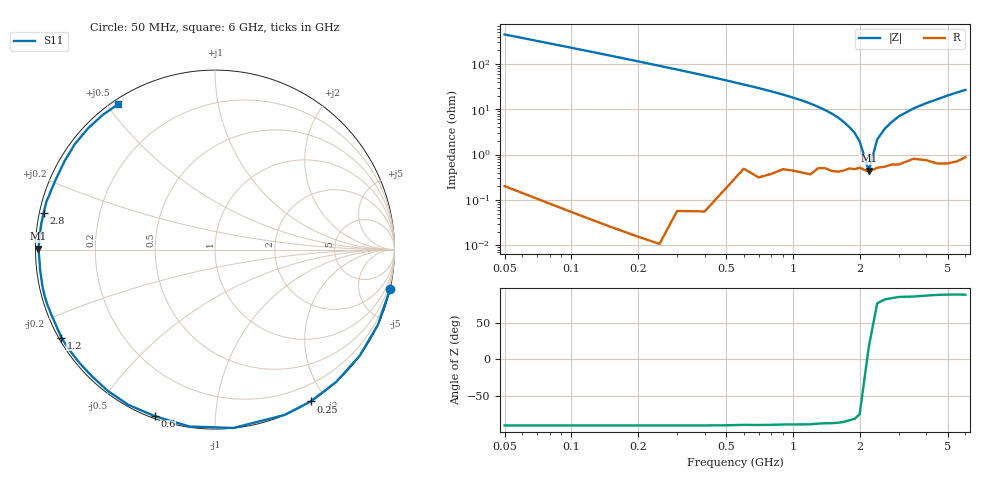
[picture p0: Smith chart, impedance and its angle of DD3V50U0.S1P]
! Infineon Technologies  Discrete & RF Semiconductors
! BBY58-02W
! Si Tuning Diode in SCD-80
! VR = 3.5 V
! S-Parameters:  June  2000
# GHz  S  MA  R  50
!  f  S11
! GHz  MAG  ANG
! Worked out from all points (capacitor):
!   34 points, 50 MHz to 6 GHz, reference 50 ohm
!   read as one part to ground: C = 6.98 pF near 50 MHz
!   lowest |Z| = 438 mohm at 2.2 GHz (marker M1)
!   series resonance near 2.187 GHz, so ESL is about 760 pH
!   S11 on the Smith chart (normalised r, x): 50 MHz: 0.00, -8.92; 250 MHz: 0.00, -1.81; 600 MHz: 0.01, -0.70; 1.2 GHz: 0.01, -0.27; 2.8 GHz: 0.01, +0.11; 6 GHz: 0.02, +0.53
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0.05  0.9999 -12.8
0.1  0.9999 -24.8
0.15  0.9999 -36.4
0.2  0.9999 -47.4
0.25  0.9999 -57.8
0.3  0.9993 -67.3
0.4  0.999 -84.1
0.5  0.9958 -98.2
0.6  0.987 -109.9
0.7  0.9907 -119.3
0.8  0.988 -127.3
0.9  0.984 -134.3
1  0.9844 -140.2
1.1  0.9855 -145.4
1.2  0.9864 -150.2
1.4  0.9809 -158.4
1.6  0.9836 -165.1
1.8  0.9805 -170.9
2.2  0.9834 179.7
2.4  0.9798 175.2
2.8  0.9763 168.0
3  0.9766 164.3
3.5  0.9695 156.5
4  0.9724 149.5
4.5  0.9775 143.0
5  0.9782 136.1
5.5  0.977 129.7
6  0.9732 123.8
